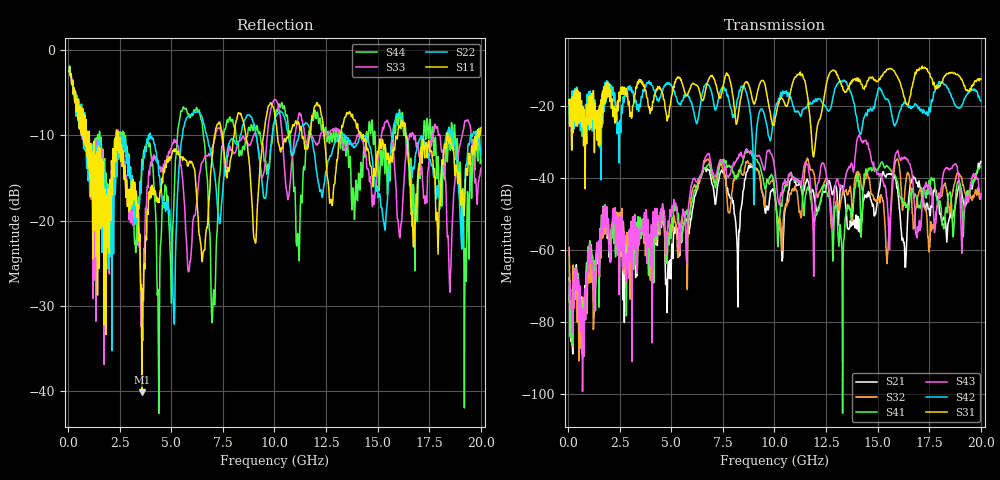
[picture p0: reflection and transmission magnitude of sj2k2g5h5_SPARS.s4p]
! FILE: E:\users\goganessyan\GBX_Backplane\FR408_backplane\1m_OUTBOUND_NEXT\sj2k2g5h5_SPARS.s4p
# MHZ S RI R 50.00
! FREQ  S11  S12  S13  S14
!  S21  S22  S23  S24
!  S31  S32  S33  S34
!  S41  S42  S43  S44
!  REAL  IMAG  REAL  IMAG  REAL  IMAG  REAL  IMAG
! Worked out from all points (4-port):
!   799 points, 50 MHz to 20 GHz, reference 50 ohm
!   strongest paths, dB at 50 MHz, 5.025 GHz, 10.03 GHz, 15.03 GHz, 20 GHz:
!     S31: -18.4, -17.1, -23.8, -13.2, -12.6
!     S42: -18.2, -14.7, -21.0, -15.4, -18.8
!     S43: -73.9, -47.8, -38.0, -38.9, -45.8
!     S41: -74.5, -51.7, -44.0, -37.4, -37.0
!     S32: -59.4, -53.0, -44.1, -46.1, -44.4
!     S21: -67.8, -58.4, -45.7, -44.9, -35.5
!   lowest |S11| = -40.2 dB at 3.575 GHz (marker M1), VSWR 1.02, Z = 49.1 + j0.328 ohm
!   |S11| at or under -10 dB: 2.43 GHz to 7.099 GHz (4.668 GHz wide, 98 % of centre); 14.3 GHz to 15.97 GHz (1.664 GHz wide, 11 % of centre); 16.36 GHz to 18.37 GHz (2.007 GHz wide, 11.6 % of centre)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
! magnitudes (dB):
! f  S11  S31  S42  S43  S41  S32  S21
! 50 MHz  -2.5  -18.4  -18.2  -73.9  -74.5  -59.4  -67.8
! 3.575 GHz  -40.2  -14.0  -17.8  -54.8  -51.6  -55.0  -51.8
! 11.9 GHz  -7.1  -34.2  -18.6  -67.4  -51.8  -38.8  -44.3
! 14.1 GHz  -9.5  -13.3  -27.1  -28.1  -40.8  -39.2  -51.4
! 15.6 GHz  -12.8  -9.7  -20.0  -55.5  -37.8  -51.5  -39.1
! 16.32 GHz  -9.2  -18.3  -19.3  -34.7  -46.8  -43.2  -64.8
! 20 GHz  -9.1  -12.6  -18.8  -45.8  -37.0  -44.4  -35.5
